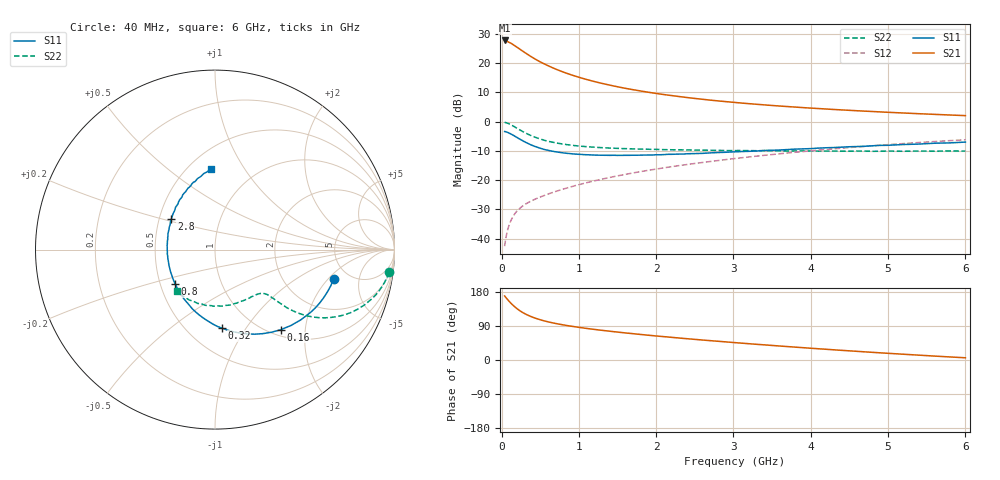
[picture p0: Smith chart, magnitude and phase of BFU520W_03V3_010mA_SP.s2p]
! Filename:  P:\Prog\Test\Noise\ATS_data\Testdata_Net\Run2\BFU520W_APM2013_06_A05_03p3V_010mA_SP_CM01_D.s2p
! Date/Time: Tue 26/Mar/2013 18:01:39
! BFU520W_APM2013_06_A05_03p3V_1to20mA_SP_CM01_Bias6_R.s2p
! MDIF S-parameter v. bias file
! BFU520W_APM2013_06_A05_03p3V_1to20mA_SP_CM01
! Date/time Tue Mar 19 16:47:37 2013
! VAR V_out= 3.3000
! VAR I_out= 9.9950
! VAR V_in= 0.8479
! VAR I_in= 0.1164
! Device data file deembeded for feedlines and parallel
! Original file: \Run2\BFU520W_APM2013_06_A05_03p3V_010mA_SP_CM01_R.s2p
! Feed-files: PR019V01_070313_Feed1.s2p, PR019V01_070313_Feed2.s2p
! Parallel-file: PR019V01_070313_Par.s2p
# MHz S MA R 50
!  Freq-MHz  S11-mag  S11-arg  S21-mag  S21-arg  S12-mag  S12-arg  S22-mag  S22-arg
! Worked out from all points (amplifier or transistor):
!   98 points, 40 MHz to 6 GHz, reference 50 ohm
!   highest |S21| = 27.8 dB at 40 MHz (marker M1)
!   |S21| within 3 dB of that: start of sweep to 238.5 MHz
!   unconditionally stable (mu >= 1): 1.35 GHz to 2.638 GHz
!   at 300 MHz: K = 0.53, MSG = 26.0 dB, |S12| = -28.4 dB
!   at 1.6 GHz: K = 1.01, MAG = 14.0 dB, |S12| = -18.0 dB
!   at 6 GHz: K = 0.87, MSG = 4.1 dB, |S12| = -6.2 dB
!   S11 on the Smith chart (normalised r, x): 40 MHz: 3.80, -2.29; 160 MHz: 1.11, -1.49; 320 MHz: 0.72, -0.78; 800 MHz: 0.60, -0.25; 2.8 GHz: 0.58, +0.22; 6 GHz: 0.64, +0.72
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40  0.6802 -13.8  24.52 169.1  0.007445 83.4  0.9777 -7.4
50  0.6764 -17.1  24.45 166.5  0.009166 82.2  0.9701 -9.2
70  0.6622 -23.8  23.74 161.6  0.01258 79.2  0.9519 -12.7
100  0.6373 -33.2  22.7 154.5  0.01733 75.4  0.9153 -17.5
120  0.6178 -39.3  22.04 150.2  0.02021 73.1  0.8885 -20.3
160  0.578 -50.4  20.38 142.4  0.02535 69.2  0.8309 -25.1
180  0.5579 -55.6  19.57 138.9  0.02759 67.8  0.8012 -27.1
220  0.5193 -65.2  18.06 132.5  0.03158 65.6  0.7462 -30.4
280  0.468 -77.7  15.9 124.6  0.0367 63.4  0.6736 -34.0
320  0.4387 -85.1  14.67 120.2  0.03969 62.6  0.6325 -35.7
400  0.3929 -97.8  12.57 113.1  0.04515 62.0  0.5663 -37.8
500  0.3529 -111.0  10.57 106.3  0.05156 62.2  0.5069 -39.0
650  0.3145 -126.7  8.488 98.5  0.06099 63.3  0.4491 -39.7
800  0.2926 -139.3  7.059 92.6  0.07061 64.5  0.4141 -40.2
1050  0.2747 -155.6  5.509 84.8  0.08714 66.1  0.3792 -41.0
1500  0.2658 -177.0  3.961 73.7  0.1185 67.1  0.3505 -44.5
2050  0.2723 164.4  2.977 62.5  0.1587 66.3  0.3351 -50.8
2800  0.2973 145.2  2.27 49.4  0.2167 63.3  0.3236 -62.8
3100  0.3089 138.6  2.088 44.6  0.2414 61.6  0.3218 -67.8
4100  0.3539 120.5  1.68 29.6  0.3265 54.8  0.3141 -87.6
5200  0.4076 103.8  1.409 15.2  0.4234 45.4  0.3123 -112.2
6000  0.4485 93.0  1.271 5.8  0.4915 37.7  0.3145 -132.2
